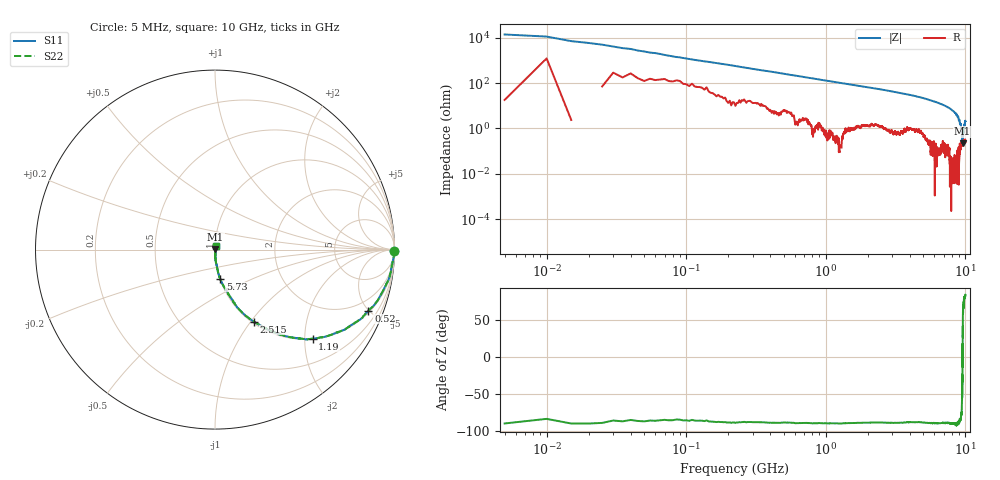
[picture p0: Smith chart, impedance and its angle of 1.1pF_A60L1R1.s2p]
! Amotech Co.,Ltd.
! http://www.amotech.co.kr/
! Part Number: A60L1R1
! These Parameters are Measured in Series Mode Connection
! Operation Temp=25[degC], DC Bias Voltage=0[V]
! Freq. Start=5[MHz] Stop=10[GHz], 2000[Steps]
! Date: Monday, July 14, 2020, 09:27:04
# GHZ S RI R 50.000000
!Freq.(Hz) S11(Real) S11(Imag) S21(Real) S21(Imag) S12(Real) S12(Imag) S22(Real) S22(Imag)
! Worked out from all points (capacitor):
!   2000 points, 5 MHz to 10 GHz, reference 50 ohm
!   read as one part in series: C = 1.3 pF near 55 MHz
!   lowest |Z| = 224 mohm at 9.545 GHz (marker M1)
!   series resonance near 9.536 GHz, so ESL is about 210 pH
!   S11 on the Smith chart (normalised r, x): 5 MHz: open; 520 MHz: 1.12, -4.97; 1.19 GHz: 1.01, -2.18; 2.515 GHz: 1.03, -1.04; 5.73 GHz: 1.01, -0.33; 10 GHz: 1.00, +0.04
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0.005  0.9999 -0.00713  6e-05 0.00713  6e-05 0.00713  0.9999 -0.00713
0.08  0.9908 -0.0642  0.00919 0.0642  0.00919 0.0642  0.9908 -0.0642
0.145  0.9815 -0.1126  0.0185 0.1126  0.0185 0.1126  0.9815 -0.1126
0.295  0.9428 -0.2164  0.0572 0.2164  0.0572 0.2164  0.9428 -0.2164
0.52  0.8548 -0.3403  0.1452 0.3403  0.1452 0.3403  0.8548 -0.3403
0.79  0.7284 -0.4407  0.2716 0.4407  0.2716 0.4407  0.7284 -0.4407
1.19  0.5437 -0.4961  0.4563 0.4961  0.4563 0.4961  0.5437 -0.4961
1.675  0.3817 -0.4782  0.6183 0.4782  0.6183 0.4782  0.3817 -0.4782
2.515  0.2183 -0.401  0.7817 0.401  0.7817 0.401  0.2183 -0.401
3.34  0.1265 -0.3248  0.8735 0.3248  0.8735 0.3248  0.1265 -0.3248
5.005  0.0494 -0.2065  0.9506 0.2065  0.9506 0.2065  0.0494 -0.2065
5.73  0.0293 -0.1611  0.9707 0.1611  0.9707 0.1611  0.0293 -0.1611
6.67  0.0158 -0.1192  0.9842 0.1192  0.9842 0.1192  0.0158 -0.1192
8.335  0.00275 -0.053  0.9973 0.053  0.9973 0.053  0.00275 -0.053
8.875  0.000618 -0.0325  0.9994 0.0325  0.9994 0.0325  0.000618 -0.0325
9.245  0.00162 -0.0157  0.9984 0.0157  0.9984 0.0157  0.00162 -0.0157
9.365  0.00188 -0.00758  0.9981 0.00758  0.9981 0.00758  0.00188 -0.00758
9.51  0.00254 -0.00171  0.9975 0.00171  0.9975 0.00171  0.00254 -0.00171
9.545  0.00213 0.000674  0.9979 -0.000674  0.9979 -0.000674  0.00213 0.000674
9.64  0.00236 0.00606  0.9976 -0.00606  0.9976 -0.00606  0.00236 0.00606
9.77  0.00265 0.0116  0.9973 -0.0116  0.9973 -0.0116  0.00265 0.0116
10  0.00283 0.0211  0.9972 -0.0211  0.9972 -0.0211  0.00283 0.0211
